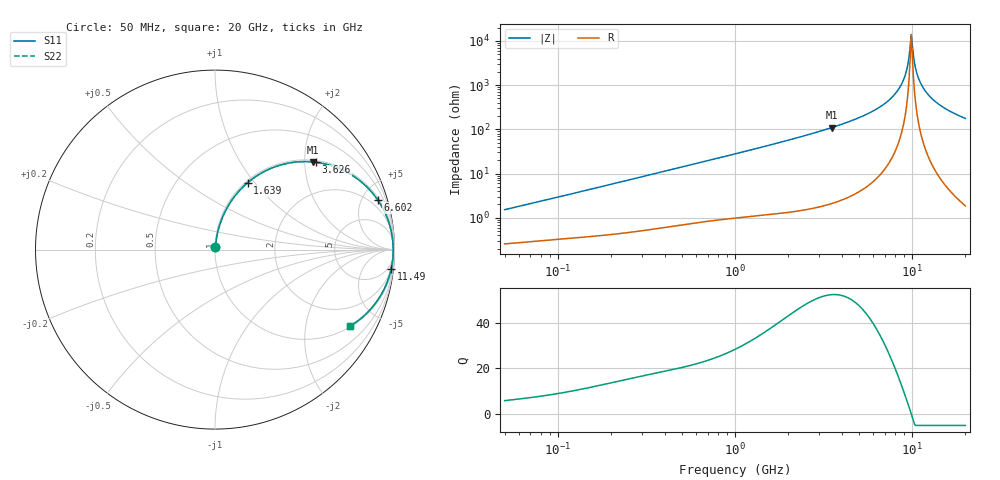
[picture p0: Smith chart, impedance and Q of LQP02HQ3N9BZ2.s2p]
!Murata Part Number: LQP02HQ3N9BZ2
!These Parameters are Measured in Series Mode Connection
!  o--[Z]--o
!Port1  Port2
!  o-------o
!Freq. Start=50[MHz] Stop=20[GHz], 401[Steps]
# Hz S RI R 50
!Freq.(Hz) S11(Real) S11(Imag) S21(Real) S21(Imag) S12(Real) S12(Imag) S22(Real) S22(Imag)
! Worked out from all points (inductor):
!   401 points, 50 MHz to 20 GHz, reference 50 ohm
!   read as one part in series: L = 4.73 nH near 51.52 MHz
!   highest Q = 52.2 at 3.519 GHz (marker M1), where L = 4.96 nH
!   self-resonance near 9.892 GHz
!   S11 on the Smith chart (normalised r, x): 50 MHz: 1.01, +0.03; 1.639 GHz: 1.02, +0.92; 3.626 GHz: 1.04, +2.28; 6.602 GHz: 1.19, +6.46; 11.49 GHz: 2, -18; 20 GHz: 1.04, -3.53
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5e7  0.00278 0.0149  0.9972 -0.0149  0.9972 -0.0149  0.00278 0.0149
1.364002e8  0.00514 0.0391  0.9949 -0.0391  0.9949 -0.0391  0.00514 0.0391
3.721004e8  0.0165 0.1027  0.9835 -0.1027  0.9835 -0.1027  0.0165 0.1027
1e9  0.0795 0.2535  0.9205 -0.2535  0.9205 -0.2535  0.0795 0.2535
1.639343e9  0.1815 0.3726  0.8185 -0.3726  0.8185 -0.3726  0.1815 0.3726
2.728004e9  0.3949 0.4788  0.6051 -0.4788  0.6051 -0.4788  0.3949 0.4788
3.519108e9  0.5451 0.4885  0.4549 -0.4885  0.4549 -0.4885  0.5451 0.4885
3.626126e9  0.5639 0.4864  0.4361 -0.4864  0.4361 -0.4864  0.5639 0.4864
5.117541e9  0.7781 0.405  0.2219 -0.405  0.2219 -0.405  0.7781 0.405
6.601595e9  0.9059 0.2777  0.0941 -0.2777  0.0941 -0.2777  0.9059 0.2777
7.442007e9  0.9487 0.2023  0.0513 -0.2023  0.0513 -0.2023  0.9487 0.2023
8.264682e9  0.9748 0.1305  0.0252 -0.1305  0.0252 -0.1305  0.9748 0.1305
8.907419e9  0.9866 0.0771  0.0134 -0.0771  0.0134 -0.0771  0.9866 0.0771
9.316812e9  0.9907 0.0445  0.00926 -0.0445  0.00926 -0.0445  0.9907 0.0445
9.745021e9  0.9928 0.0117  0.00725 -0.0117  0.00725 -0.0117  0.9928 0.0117
9.892087e9  0.9929 0.000717  0.00707 -0.000717  0.00707 -0.000717  0.9929 0.000717
1.019291e10  0.9926 -0.0212  0.00743 0.0212  0.00743 0.0212  0.9926 -0.0212
1.066139e10  0.9902 -0.054  0.0098 0.054  0.0098 0.054  0.9902 -0.054
1.149051e10  0.9814 -0.1081  0.0186 0.1081  0.0186 0.1081  0.9814 -0.1081
1.257102e10  0.9631 -0.1712  0.0369 0.1712  0.0369 0.1712  0.9631 -0.1712
1.417136e10  0.926 -0.2503  0.074 0.2503  0.074 0.2503  0.926 -0.2503
2e10  0.7549 -0.4249  0.2451 0.4249  0.2451 0.4249  0.7549 -0.4249
